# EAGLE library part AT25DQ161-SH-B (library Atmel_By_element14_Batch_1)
SPI Serial Flash
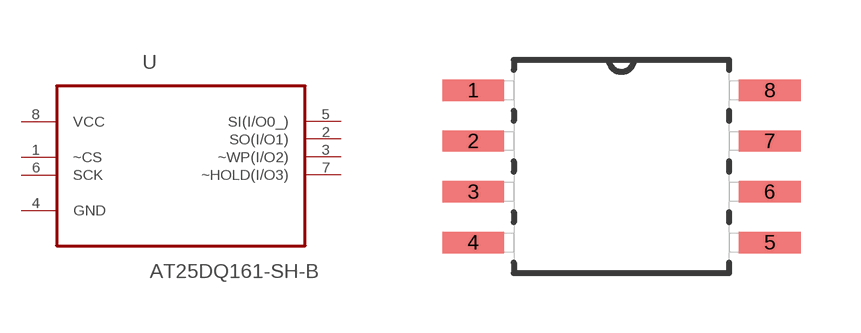
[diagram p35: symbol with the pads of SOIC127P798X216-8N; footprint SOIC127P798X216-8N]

Designator prefix U

## AT25DQ161-SH-B (MPN: AT25DQ161-SH-B; OC_FARNELL: 1841584; OC_NEWARK: 12T1350; PACKAGE: SOIC-8; SUPPLIER: Atmel)  [SOIC127P798X216-8N]
1  ~CS  in
2  SO(I/O1)
3  ~WP(I/O2)
4  GND  pas
5  SI(I/O0_)
6  SCK  in
7  ~HOLD(I/O3)
8  VCC  pwr

## Footprint SOIC127P798X216-8N (pad centres in mm)
smd 1.549 x 0.533: 1 -3.708,1.905; 2 -3.708,0.635; 3 -3.708,-0.635; 4 -3.708,-1.905; 5 3.708,-1.905; 6 3.708,-0.635; 7 3.708,0.635; 8 3.708,1.905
